TYPE ST_EL5131_OUTPUT :
STRUCT
	{attribute 'displaymode':='bin'}
	Control							:	ST_Control_UINT_TO_BIT;
	Set_counter_value				:	UDINT;
	Contro_OutputChn1				:	ST_ENC_Control_Output_Channel;
	Contro_OutputChn2				:	ST_ENC_Control_Output_Channel;
END_STRUCT
END_TYPE
